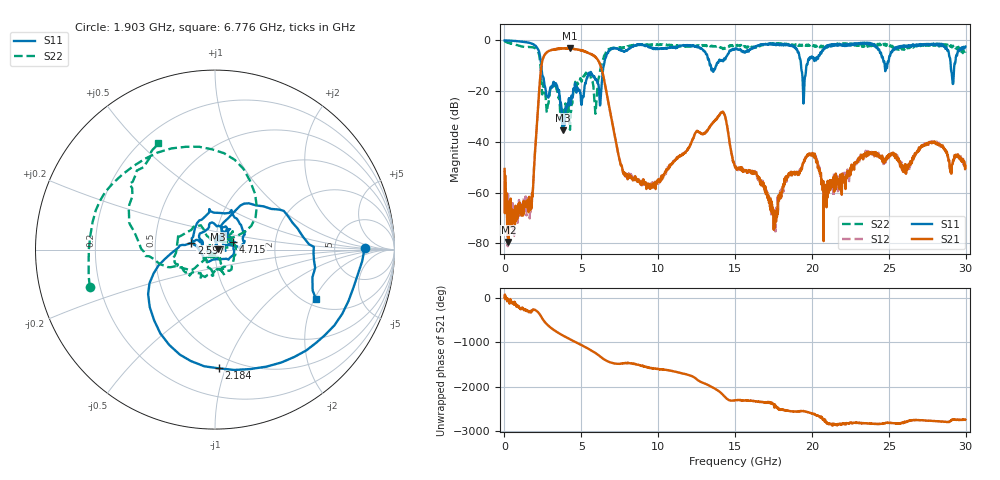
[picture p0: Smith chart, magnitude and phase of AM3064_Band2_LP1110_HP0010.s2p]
# Hz S DB R 50.0
!freq dBS11 angS11 dBS21 angS21 dBS12 angS12 dBS22 angS22
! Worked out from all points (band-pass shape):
!   1600 points, 10 MHz to 29.98 GHz, reference 50 ohm
!   highest |S21| = -3.10 dB at 4.246 GHz (marker M1); lowest = -79.4 dB at 253.7 MHz (marker M2)
!   |S21| within 3 dB of the highest: 2.578 GHz to 5.833 GHz (3.255 GHz wide, 77.4 % of centre)
!   lowest |S11| = -35.5 dB at 3.815 GHz (marker M3), VSWR 1.03, Z = 51.7 + j0.155 ohm
!   |S11| at or under -10 dB: 2.395 GHz to 6.454 GHz (4.059 GHz wide, 91.7 % of centre); 13.42 GHz to 13.76 GHz (336 MHz wide, 2.47 % of centre); 19.29 GHz to 19.64 GHz (348.1 MHz wide, 1.79 % of centre)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
!   |S22| runs from -35.2 to -0.3 dB; largest |S21 - S12| = 0.02
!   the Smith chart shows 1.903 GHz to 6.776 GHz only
!   S11 on the Smith chart (normalised r, x): 1.903 GHz: 11, +1; 2.184 GHz: 0.40, -0.95; 2.597 GHz: 0.77, +0.06; 4.715 GHz: 1.22, +0.10; 6.776 GHz: 2.28, -2.06
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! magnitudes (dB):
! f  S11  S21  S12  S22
! 10 MHz  0.0  -50.7  -51.2  -0.3
! 253.7 MHz  -0.1  -79.4  -70.9  -1.0
! 1.622 GHz  -1.0  -65.3  -65.7  -2.6
! 1.903 GHz  -1.6  -52.9  -52.3  -2.8
! 2.184 GHz  -3.6  -26.1  -26.1  -4.5
! 2.597 GHz  -17.3  -5.9  -5.8  -19.1
! 3.815 GHz  -35.5  -3.1  -3.1  -30.1
! 4.246 GHz  -23.4  -3.1  -3.2  -34.6
! 4.715 GHz  -19.3  -3.6  -3.6  -17.5
! 5.015 GHz  -25.4  -4.0  -4.0  -16.3
! 5.933 GHz  -15.7  -6.7  -6.6  -28.0
! 6.776 GHz  -4.1  -25.1  -24.8  -3.4
! 7.77 GHz  -4.4  -52.7  -52.4  -2.9
! 10 GHz  -3.3  -55.8  -55.9  -1.8
! 14.14 GHz  -7.8  -28.2  -28.2  -2.9
! 15 GHz  -3.3  -50.1  -49.8  -2.0
! 17.61 GHz  -1.7  -68.3  -66.6  -1.1
! 19.47 GHz  -24.1  -48.2  -47.5  -2.2
! 19.99 GHz  -6.4  -45.1  -45.0  -1.7
! 20.85 GHz  -3.1  -61.9  -59.8  -2.4
! 25 GHz  -8.0  -45.0  -46.0  -1.7
! 29.98 GHz  -2.5  -49.3  -50.7  -4.5
